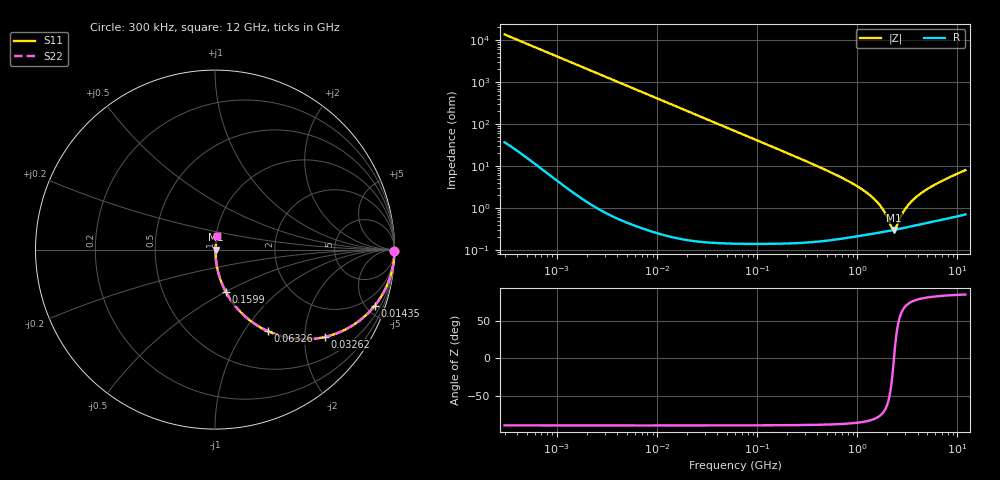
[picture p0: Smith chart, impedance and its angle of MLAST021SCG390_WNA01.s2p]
! MLAST021SCG390_WNA01  S-PARAMETER MODEL  ( Standard Model )
! Model Generated by TAIYO YUDEN Corporation (http://www.ty-top.com)
! Version 2.0
! TAIYO YUDEN Control No. 231201
! Copyright(c) 2023 TAIYO YUDEN CO.,LTD. All Rights Reserved.
! Product Description (link to TY-COMPAS)
! https://ds.yuden.co.jp/TYCOMPAS/or/detail?pn=MLAST021SCG390JWNA01&u=M
! Products Name : Multilayer Ceramic Capacitors
! Characteristics :
!  Capacitance : 39 [pF] , Rated Voltage : 25 [V] , TCC : CG / C0G
!  Case Size : 0.25 x 0.125 / 0.0098 x 0.0049 [mm/inch] , Thickness : 0.125 / 0.0049 [mm/inch]
!  (Conditions: Temperature = 25 [degC] , DC Bias Voltage = 0 [V])
! External Node Assignments :
!  1  o---| |---o  2
! GND o---------o GND
! Frequency Range : 0.3MHz  -  12000MHz  [ 401 STEP ]
# MHZ S RI R 50
! Freq[MHz].  S11 Real  S11 Imag  S21 Real  S21 Imag  S12 Real  S12 Imag  S22 Real  S22 Imag
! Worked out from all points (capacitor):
!   401 points, 300 kHz to 12 GHz, reference 50 ohm
!   read as one part in series: C = 39 pF near 316.3 kHz
!   lowest |Z| = 300 mohm at 2.322 GHz (marker M1)
!   series resonance near 2.322 GHz, so ESL is about 120 pH
!   S11 on the Smith chart (normalised r, x): 300 kHz: open; 14.35 MHz: 1.00, -5.70; 32.62 MHz: 1.00, -2.51; 63.26 MHz: 1.00, -1.29; 159.9 MHz: 1.00, -0.51; 12 GHz: 1.01, +0.16
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0.3  0.9999 -0.00735  7.39e-05 0.00735  7.39e-05 0.00735  0.9999 -0.00735
1.769972  0.9981 -0.0432  0.0019 0.0432  0.0019 0.0432  0.9981 -0.0432
4.716902  0.9868 -0.1139  0.0132 0.1139  0.0132 0.1139  0.9868 -0.1139
10.44266  0.9386 -0.2397  0.0614 0.2397  0.0614 0.2397  0.9386 -0.2397
14.3507  0.8901 -0.3124  0.1099 0.3124  0.1099 0.3124  0.8901 -0.3124
32.62367  0.6107 -0.487  0.3893 0.487  0.3893 0.487  0.6107 -0.487
60  0.3171 -0.4643  0.6829 0.4643  0.6829 0.4643  0.3171 -0.4643
63.26471  0.2946 -0.4548  0.7054 0.4548  0.7054 0.4548  0.2946 -0.4548
99.25425  0.1454 -0.3508  0.8546 0.3508  0.8546 0.3508  0.1454 -0.3508
159.8975  0.0619 -0.2382  0.9381 0.2382  0.9381 0.2382  0.0619 -0.2382
353.9943  0.014 -0.1107  0.986 0.1107  0.986 0.1107  0.014 -0.1107
763.2128  0.00413 -0.047  0.9959 0.047  0.9959 0.047  0.00413 -0.047
1229.528  0.00284 -0.0234  0.9972 0.0234  0.9972 0.0234  0.00284 -0.0234
1689.663  0.00272 -0.011  0.9973 0.011  0.9973 0.011  0.00272 -0.011
2088.533  0.00286 -0.00361  0.9971 0.00361  0.9971 0.00361  0.00286 -0.00361
2202.174  0.00292 -0.0018  0.9971 0.0018  0.9971 0.0018  0.00292 -0.0018
2321.999  0.00299 3.1e-08  0.997 -3.1e-08  0.997 -3.1e-08  0.00299 3.1e-08
2448.343  0.00307 0.00179  0.9969 -0.00179  0.9969 -0.00179  0.00307 0.00179
3026.31  0.00348 0.00899  0.9965 -0.00899  0.9965 -0.00899  0.00348 0.00899
3944.255  0.00423 0.0184  0.9958 -0.0184  0.9958 -0.0184  0.00423 0.0184
6188.031  0.00628 0.0371  0.9937 -0.0371  0.9937 -0.0371  0.00628 0.0371
12000  0.0131 0.0778  0.9869 -0.0778  0.9869 -0.0778  0.0131 0.0778
